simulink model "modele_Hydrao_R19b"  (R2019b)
settings: Solver=VariableStepAuto  StartTime=0.0  StopTime=1  MaxStep=2e-4  RelTol=1e-3
libraries: fl_lib x9, nesl_utility x3

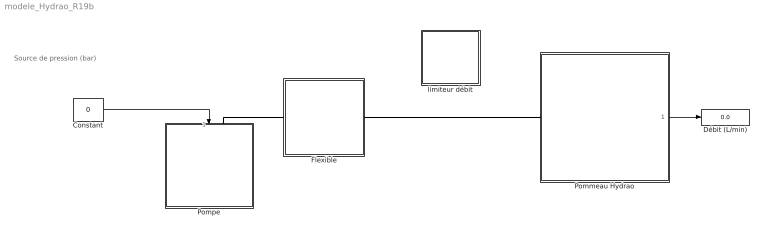
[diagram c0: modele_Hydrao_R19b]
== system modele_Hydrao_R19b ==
  note: Source de pression (bar)
  Constant : Constant  Value=0
  Débit (L/min) : Display
  Flexible : Subsystem
  Pommeau Hydrao : Subsystem
  Pompe : Subsystem
  limiteur débit : Subsystem
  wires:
  Constant/1 -> Pompe/1(In1)
  Pommeau Hydrao/1(Out1) -> Débit (L/min)/1
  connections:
  Flexible/RConn1 -- Pommeau Hydrao/LConn1
  Pompe/LConn1 -- Flexible/LConn1

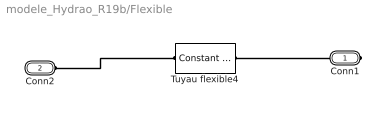
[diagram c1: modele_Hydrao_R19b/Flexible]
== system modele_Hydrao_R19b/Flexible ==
  Tuyau flexible4 : fl_lib/Hydraulic/Hydraulic Elements/Constant Area Hydraulic Orifice  area=41e-6 m^2  C_d=0.251  lam_spec=2  B_lam=2000  Re_cr=1e0  q_specify=off  q_priority=None  q=0.001 m^3/s  q_nominal_specify=off  q_nominal_unit=m^3/s  q_nominal_value=1  p_specify=off  p_priority=None  p=0 Pa  p_nominal_specify=off  p_nominal_unit=Pa  p_nominal_value=1
  Conn1 : PMIOPort  Side=Right
  Conn2 : PMIOPort  Port=2  Side=Left
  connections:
  Conn2/RConn1 -- Tuyau flexible4/LConn1
  Tuyau flexible4/RConn1 -- Conn1/RConn1

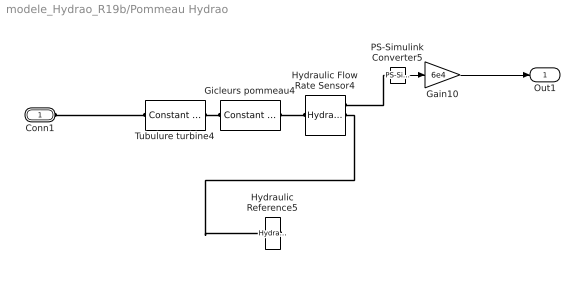
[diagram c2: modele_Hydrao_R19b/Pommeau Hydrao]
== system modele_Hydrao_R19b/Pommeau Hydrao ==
  Gain10 : Gain  Gain=6e4
  Gicleurs pommeau4 : fl_lib/Hydraulic/Hydraulic Elements/Constant Area Hydraulic Orifice  area=20e-6 m^2  C_d=0.4  lam_spec=2  B_lam=0.999  Re_cr=1e0  q_specify=off  q_priority=None  q=0.001 m^3/s  q_nominal_specify=off  q_nominal_unit=m^3/s  q_nominal_value=1  p_specify=off  p_priority=None  p=0 Pa  p_nominal_specify=off  p_nominal_unit=Pa  p_nominal_value=1
  Hydraulic Flow Rate Sensor4 : fl_lib/Hydraulic/Hydraulic Sensors/Hydraulic Flow Rate Sensor
  Hydraulic Reference5 : fl_lib/Hydraulic/Hydraulic Elements/Hydraulic Reference
  PS-Simulink Converter5 : nesl_utility/PS-Simulink Converter  PhysicalDomain=network_engine_domain  SubClassName=ps_output  LeftPortType=input  RightPortType=output  PseudoPeriodic=off  Frequencies=[]  Unit=inherit  AffineConversion=off
  Tubulure turbine4 : fl_lib/Hydraulic/Hydraulic Elements/Constant Area Hydraulic Orifice  area=12.7e-6 m^2  C_d=0.81  lam_spec=2  B_lam=0.999  Re_cr=1e0  q_specify=off  q_priority=None  q=0.001 m^3/s  q_nominal_specify=off  q_nominal_unit=m^3/s  q_nominal_value=1  p_specify=off  p_priority=None  p=0 Pa  p_nominal_specify=off  p_nominal_unit=Pa  p_nominal_value=1
  Conn1 : PMIOPort  Side=Left
  Out1 : Outport
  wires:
  PS-Simulink Converter5/1 -> Gain10/1
  Gain10/1 -> Out1/1
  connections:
  PS-Simulink Converter5/LConn1 -- Hydraulic Flow Rate Sensor4/RConn1
  Conn1/RConn1 -- Tubulure turbine4/LConn1
  Gicleurs pommeau4/LConn1 -- Tubulure turbine4/RConn1
  Gicleurs pommeau4/RConn1 -- Hydraulic Flow Rate Sensor4/LConn1
  Hydraulic Flow Rate Sensor4/RConn2 -- Hydraulic Reference5/LConn1

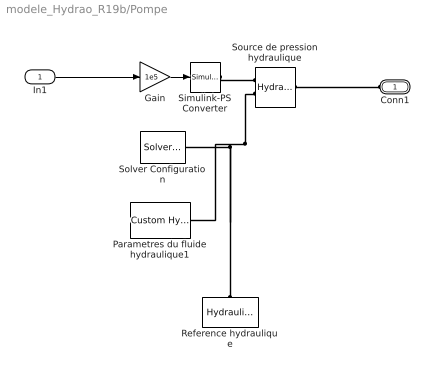
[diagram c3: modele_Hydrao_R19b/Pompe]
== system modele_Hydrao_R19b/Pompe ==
  In1 : Inport
  Gain : Gain  Gain=1e5
  Parametres du fluide hydraulique1 : fl_lib/Hydraulic/Hydraulic Utilities/Custom Hydraulic Fluid  density=994 kg/m^3  viscosity_kin=7.35e-7 m^2/s  bulk=8e8 Pa  alpha=0.005  range_error=2
  Reference hydraulique : fl_lib/Hydraulic/Hydraulic Elements/Hydraulic Reference
  Simulink-PS Converter : nesl_utility/Simulink-PS Converter  PhysicalDomain=network_engine_domain  SubClassName=ps_input  LeftPortType=input  RightPortType=output  PseudoPeriodic=off  Frequencies=[]  NoiseDistribution=none  NoiseParameters=[]  Unit=1  AffineConversion=off  FilteringAndDerivatives=provide  SimscapeFilterOrder=1  InputFilterTimeConstant=0.001  UdotUserProvided=0
  Solver Configuration : nesl_utility/Solver Configuration  PhysicalDomain=network_engine_domain  SubClassName=solver  LeftPortType=input  RightPortType=generic  Tones=[]  Harmonics=[]  SimulateNoise=off  Profile=off  UseLocalSampling=off  EnableSwitchedLinearOptims=on  FrequencyDomain=off  UseCCode=off  RelTol=0.001  AbsTol=1e-06  MinStep=1e-09  ToWorkspace=off  RevertToSquareIcSolve=off  NumHomotopyIterations=100  PhasorMode=off  PhasorModeNumHarmonics=1  DoDC=off  ResidualTolerance=1e-9  UseLocalSolver=off  LocalSolverChoice=NE_BACKWARD_EULER_ADVANCER  LocalSolverSampleTime=0.001  DoFixedCost=off  MaxNonlinIter=3  MaxModeIter=2  LinearAlgebra=Sparse  EquationFormulation=NE_TIME_EF  DelaysMemoryBudget=1024  AutomaticFiltering=on  FilteringTimeConstant=0.001  PartitionStorageMethod=AS_NEEDED  PartitionMemoryBudget=1024  PartitionMethod=FAST
  Source de pression hydraulique : fl_lib/Hydraulic/Hydraulic Sources/Hydraulic Pressure Source
  Conn1 : PMIOPort  Side=Left
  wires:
  Gain/1 -> Simulink-PS Converter/1
  In1/1 -> Gain/1
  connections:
  Source de pression hydraulique/LConn1 -- Conn1/RConn1
  Source de pression hydraulique/RConn2 -- Parametres du fluide hydraulique1/RConn1 -- Reference hydraulique/LConn1 -- Solver Configuration/RConn1
  Simulink-PS Converter/RConn1 -- Source de pression hydraulique/RConn1

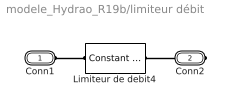
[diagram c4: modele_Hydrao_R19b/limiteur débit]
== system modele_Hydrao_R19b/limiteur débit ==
  Limiteur de debit4 : fl_lib/Hydraulic/Hydraulic Elements/Constant Area Hydraulic Orifice  area=20e-6 m^2  C_d=0.5  lam_spec=2  B_lam=0.999  Re_cr=1e0  q_specify=off  q_priority=None  q=0.001 m^3/s  q_nominal_specify=off  q_nominal_unit=m^3/s  q_nominal_value=1  p_specify=off  p_priority=None  p=0 Pa  p_nominal_specify=off  p_nominal_unit=Pa  p_nominal_value=1
  Conn1 : PMIOPort  Side=Left
  Conn2 : PMIOPort  Port=2  Side=Right
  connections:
  Limiteur de debit4/RConn1 -- Conn2/RConn1
  Limiteur de debit4/LConn1 -- Conn1/RConn1
